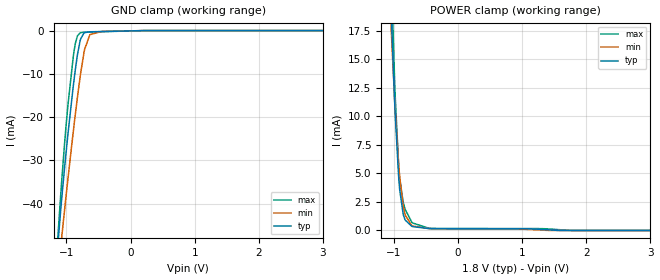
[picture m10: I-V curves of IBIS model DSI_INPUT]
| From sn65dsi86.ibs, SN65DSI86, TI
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|   Model
[Model]   DSI_INPUT
Model_type   Input
Vinl = 0.54
Vinh = 1.26
|   typ   min   max
C_comp   1.577pF   1.508pF   1.625pF
[Voltage Range]   1.8   1.65   1.98
[Temperature Range]   27   125   -40
[Power Clamp Reference]   1.8   1.65   1.98
[GND Clamp Reference]   -0   -0   -0
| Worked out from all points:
|   GND clamp passes 1 mA (typ) near -0.74 V on its own axis
|   POWER clamp passes 1 mA (typ) near -0.83 V on its own axis
[GND Clamp]
|   Voltage   I(typ)   I(min)   I(max)
-1.8V     -204.9mA   -194mA     -215.8mA
-1.141V   -51.17mA   -57.85mA   -49.71mA
-1.087V   -41.36mA   -49.89mA   -37.86mA
-1.071V   -38.63mA   -47.57mA   -34.49mA
-984.6mV  -25.33mA   -35.57mA   -18.71mA
-892.8mV  -12.94mA   -23.46mA   -6.094mA
-828mV    -5.648mA   -15.5mA    -1.258mA
-784.8mV  -2.294mA   -10.65mA   -536uA
-714.6mV  -472uA     -4.298mA   -369.2uA
-633.6mV  -286.7uA   -945.5uA   -332.1uA
-450mV    -218.6uA   -199.5uA   -260.5uA
3.595V    0A         0A         0A
[POWER Clamp]
|   Voltage   I(typ)   I(min)   I(max)
-1.8V     177.3mA    144.8mA    213.6mA
-1.044V   19.54mA    18mA       23.36mA
-1.039V   18.67mA    17.32mA    22.29mA
-990mV    11.56mA    11.68mA    13.48mA
-979.2mV  10.17mA    10.55mA    11.81mA
-925.2mV  4.685mA    5.805mA    5.647mA
-909mV    3.572mA    4.706mA    4.55mA
-855mV    1.439mA    2.169mA    2.496mA
-828mV    976.4uA    1.456mA    1.933mA
-720mV    363.9uA    423.1uA    720.8uA
-406.8mV  159.4uA    157.3uA    185.2uA
3.595V    0A         0A         0A
